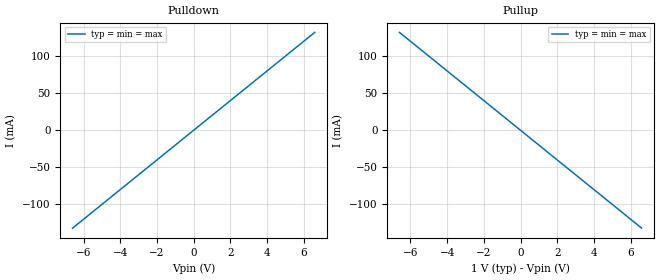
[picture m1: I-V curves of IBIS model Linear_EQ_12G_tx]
|Texas Instruments Incorporated
|Low Power 12.5 Gbps Linear Repeater
| Marketing part#   Voltage Range   Package-type   #pins
| DS125BR820NJYR/T   2.375to  3.6V   WQFN   54
| DS125BR111RTWR/T   2.375to  3.6V   RTW   24
| DS80PCI810NJYR/T   2.375to  3.6V   WQFN   54
| DS125BR401ANJYR/T   2.375to  3.6V   WQFN   54
[IBIS Ver]   5.0
[File Name]   linear_eq_12g.ibs
[File Rev]   2.0
[Date]   04/29/2024
[Source]   Texas Instruments Incorporated.
|   Analog-eLab, HPA
|   12500 TI Blvd
|   Dallas, TX -75243
|   For Support e-mail: elab_ibis@list.ti.com
[Notes]
 -Revision History:
 1.0: 8/24/2014
 - Initial version of the model
 2.0: 4/29/2024
 - Updated documentation for public release.
[Disclaimer]
 This product is designed as an aid for customers of Texas Instruments.
 No warranties, either expressed or implied, with respect to this third
 party software (if any) or with respect to its fitness for any
 particular purpose is claimed by Texas Instruments or the author. The
 software (if any) is provided solely on an "as is" basis. The entire
 risk as to its quality and performance is with the customer
[Copyright] (C) Copyright 2012 Texas Instruments Incorporated.
   All rights reserved.
|   Component  Linear_EQ_12G
[Component]   Linear_EQ_12G
[Manufacturer] Texas Instruments Incorporated
[Package]
R_pkg  0.0   NA   NA
L_pkg  0.0   NA   NA
C_pkg  0.0   NA   NA
[Pin]   signal_name   model_name   R_pin L_pin  C_pin
2p   Linear_EQ_12G_rx_2p   Linear_EQ_12G_rx
2n   Linear_EQ_12G_rx_2n   Linear_EQ_12G_rx
1p   Linear_EQ_12G_tx_p   Linear_EQ_12G_tx
1n   Linear_EQ_12G_tx_n   Linear_EQ_12G_tx
[Diff_Pin] inv_pin vdiff tdelay_typ tdelay_min tdelay_max
2p   2n   NA   NA   NA   NA
1p   1n   NA   NA   NA   NA
[Model] Linear_EQ_12G_rx
Model_type Input
C_comp 0p 0p 0p
Vinh = 0.7
Vinl = 0.3
[Temperature_Range] 25 125 0
[Voltage Range] 1.0 1.0 1.0
[Algorithmic Model]
Executable Windows_cl16.00.30319.01_64 Linear_EQ_12G_rx_x64.dll Linear_EQ_12G_rx.ami
Executable Windows_cl16.00.30319.01_32 Linear_EQ_12G_rx.dll Linear_EQ_12G_rx.ami
Executable Linux_gcc4.7.2_64 Linear_EQ_12G_rx_x64.so Linear_EQ_12G_rx.ami
[End Algorithmic Model]
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| Models and submodels in the file (2): Linear_EQ_12G_tx (Output), Linear_EQ_12G_rx (Input)
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[Model] Linear_EQ_12G_tx
Model_type Output
C_comp 0p 0p 0p
Cref = 0
Vref = 0.5
Rref = 50
Vmeas = 0.5
[Temperature_Range] 25 125 0
[Voltage Range] 1.0 1.0 1.0
[Algorithmic Model]
Executable Windows_cl16.00.30319.01_64 Linear_EQ_12G_tx_x64.dll Linear_EQ_12G_tx.ami
Executable Windows_cl16.00.30319.01_32 Linear_EQ_12G_tx.dll Linear_EQ_12G_tx.ami
Executable Linux_gcc4.7.2_64 Linear_EQ_12G_tx_x64.so Linear_EQ_12G_tx.ami
[End Algorithmic Model]
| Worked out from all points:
|   slope of the pulldown table from 0 to 0.15 V, typ, clamps not added: 50 ohm
|   slope of the pullup table from 0 to 0.15 V, typ, clamps not added: 50 ohm
[Pulldown]
-6.6V     -132mA     -132mA     -132mA
0V        0A         0A         0A
6.6V      132mA      132mA      132mA
[Pullup]
-6.6V     132mA      132mA      132mA
0V        0A         0A         0A
6.6V      -132mA     -132mA     -132mA
[GND Clamp]
-6.6V     0A         0A         0A
0V        0A         0A         0A
6.6V      0A         0A         0A
[Power Clamp]
-6.6V     0A         0A         0A
0V        0A         0A         0A
6.6V      0A         0A         0A
[Ramp]
dV/dt_r 1.0/5p 1.0/5p 1.0/5p
dV/dt_f 1.0/5p 1.0/5p 1.0/5p
